TYPE "Warnungen"
TITLE =Warnmeldungen
AUTHOR : dfb
FAMILY : Meld
NAME : WarnMeld
VERSION : 0.1


  STRUCT
    Anzahl_Meldeworte : INT  := 12; // Anzahl Warnmeldeworte
HZ01 : STRUCT //Heizzone 01 Warnmeldungen 1-16
W001_HZ01_Brn_1_Stoer : Bool ;  //W001: Zone 1 Brenner 1 Brennerstörung
W002_HZ01_Brn_2_Stoer : Bool ;  //W002: Zone 1 Brenner 2 Brennerstörung
W003_HZ01_Brn_3_Stoer : Bool ;  //W003: Zone 1 Brenner 3 Brennerstörung
W004_HZ01_Brn_4_Stoer : Bool ;  //W004: Zone 1 Brenner 4 Brennerstörung
W005_HZ01_Brn_5_Stoer : Bool ;  //W005: Zone 1 Brenner 5 Brennerstörung
W006 : Bool ;  //W006:
W007 : Bool ;  //W007:
W008 : Bool ;  //W008:
W009 : Bool ;  //W009:
W010 : Bool ;  //W010:
W011 : Bool ;  //W011:
W012 : Bool ;  //W012:
W013 : Bool ;  //W013:
W014 : Bool ;  //W014:
W015 : Bool ;  //W015:
W016 : Bool ;  //W016:
END_STRUCT ;
HZ02 : STRUCT //Heizzone 02 Warnmeldungen 17-32
W017_HZ02_Brn_1_Stoer : Bool ;  //W017: Zone 2 Brenner 1 Brennerstörung
W018_HZ02_Brn_2_Stoer : Bool ;  //W018: Zone 2 Brenner 2 Brennerstörung
W019_HZ02_Brn_3_Stoer : Bool ;  //W019: Zone 2 Brenner 3 Brennerstörung
W020_HZ02_Brn_4_Stoer : Bool ;  //W020: Zone 2 Brenner 4 Brennerstörung
W021 : Bool ;  //W021:
W022 : Bool ;  //W022:
W023 : Bool ;  //W023:
W024 : Bool ;  //W024:
W025 : Bool ;  //W025:
W026 : Bool ;  //W026:
W027 : Bool ;  //W027:
W028 : Bool ;  //W028:
W029 : Bool ;  //W029:
W030 : Bool ;  //W030:
W031 : Bool ;  //W031:
W032 : Bool ;  //W032:
END_STRUCT ;
HZ03 : STRUCT //Heizzone 03 Warnmeldungen 33-48
W033_HZ03_Brn_1_Stoer : Bool ;  //W033: Zone 3 Brenner 1 Brennerstörung
W034_HZ03_Brn_2_Stoer : Bool ;  //W034: Zone 3 Brenner 2 Brennerstörung
W035_HZ03_Brn_3_Stoer : Bool ;  //W035: Zone 3 Brenner 3 Brennerstörung
W036 : Bool ;  //W036:
W037 : Bool ;  //W037:
W038 : Bool ;  //W038:
W039 : Bool ;  //W039:
W040 : Bool ;  //W040:
W041 : Bool ;  //W041:
W042 : Bool ;  //W042:
W043 : Bool ;  //W043:
W044 : Bool ;  //W044:
W045 : Bool ;  //W045:
W046 : Bool ;  //W046:
W047 : Bool ;  //W047:
W048 : Bool ;  //W048:
END_STRUCT ;
HZ04 : STRUCT //Heizzone 04 Warnmeldungen 49-64
W049_HZ04_Brn_1_Stoer : Bool ;  //W049: Zone 4 Brenner 1 Brennerstörung
W050_HZ04_Brn_2_Stoer : Bool ;  //W050: Zone 4 Brenner 2 Brennerstörung
W051 : Bool ;  //W051:
W052 : Bool ;  //W052:
W053 : Bool ;  //W053:
W054 : Bool ;  //W054:
W055 : Bool ;  //W055:
W056 : Bool ;  //W056:
W057 : Bool ;  //W057:
W058 : Bool ;  //W058:
W059 : Bool ;  //W059:
W060 : Bool ;  //W060:
W061 : Bool ;  //W061:
W062 : Bool ;  //W062:
W063 : Bool ;  //W063:
W064 : Bool ;  //W064:
END_STRUCT ;
HZ05 : STRUCT //Heizzone 05 Warnmeldungen 65-80
W065_HZ05_Brn_1_Stoer : Bool ;  //W065: Zone 5 Brenner 1 Brennerstörung
W066_HZ05_Brn_2_Stoer : Bool ;  //W066: Zone 5 Brenner 2 Brennerstörung
W067 : Bool ;  //W067:
W068 : Bool ;  //W068:
W069 : Bool ;  //W069:
W070 : Bool ;  //W070:
W071 : Bool ;  //W071:
W072 : Bool ;  //W072:
W073 : Bool ;  //W073:
W074 : Bool ;  //W074:
W075 : Bool ;  //W075:
W076 : Bool ;  //W076:
W077 : Bool ;  //W077:
W078 : Bool ;  //W078:
W079 : Bool ;  //W079:
W080 : Bool ;  //W080:
END_STRUCT ;
HZ06 : STRUCT //Heizzone 06 Warnmeldungen 81-96
W081_HZ06_Brn_1_Stoer : Bool ;  //W081: Zone 6 Brenner 1 Brennerstörung
W082_HZ06_Brn_2_Stoer : Bool ;  //W082: Zone 6 Brenner 2 Brennerstörung
W083_HZ06_Brn_3_Stoer : Bool ;  //W083: Zone 6 Brenner 3 Brennerstörung
W084 : Bool ;  //W084:
W085 : Bool ;  //W085:
W086 : Bool ;  //W086:
W087 : Bool ;  //W087:
W088 : Bool ;  //W088:
W089 : Bool ;  //W089:
W090 : Bool ;  //W090:
W091 : Bool ;  //W091:
W092 : Bool ;  //W092:
W093 : Bool ;  //W093:
W094 : Bool ;  //W094:
W095 : Bool ;  //W095:
W096 : Bool ;  //W096:
END_STRUCT ;
HZ07 : STRUCT //Heizzone 07 Warnmeldungen 97-112
W097_HZ07_Brn_1_Stoer : Bool ;  //W097: Zone 7 Brenner 1 Brennerstörung
W098_HZ07_Brn_2_Stoer : Bool ;  //W098: Zone 7 Brenner 2 Brennerstörung
W099 : Bool ;  //W099:
W100 : Bool ;  //W100:
W101 : Bool ;  //W101:
W102 : Bool ;  //W102:
W103 : Bool ;  //W103:
W104 : Bool ;  //W104:
W105 : Bool ;  //W105:
W106 : Bool ;  //W106:
W107 : Bool ;  //W107:
W108 : Bool ;  //W108:
W109 : Bool ;  //W109:
W110 : Bool ;  //W110:
W111 : Bool ;  //W111:
W112 : Bool ;  //W112:
END_STRUCT ;
NA_SK: STRUCT //Not Aus und Schutzkreise Meldungen 113-128
W113_Not_Aus_OE_ausgel : Bool ;  //W113: Not Aus hat ausgelöst
W114_Schkr_Ofeneinl : Bool ;  //W114: Schutzkreis Ofeneinlauf nicht geschlossen
W115_Schkr_Ofenausl : Bool ;  //W115: Schutzkreis Ofenauslauf nicht geschlossen
W116_NA_Tast_Ofeneinl : Bool ;  //W116: Not Aus Taster Bedienpult Ofeneinlauf betätigt
W117_NA_Tast_Ofenausl : Bool ;  //W117: Not Aus Taster Bedienpult Ofenauslauf betätigt
W118 : Bool ;  //W118:
W119 : Bool ;  //W119:
W120 : Bool ;  //W120:
W121 : Bool ;  //W121:
W122 : Bool ;  //W122:
W123 : Bool ;  //W123:
W124 : Bool ;  //W124:
W125 : Bool ;  //W125:
W126 : Bool ;  //W126:
W127 : Bool ;  //W127:
W128 : Bool ;  //W128:
END_STRUCT ;
Netz : STRUCT  //Versorgungsnetz Meldungen 129-144
W129_Q_Notnetz_niO : Bool ;  //W129: Hauptschalter Notnetz nicht eingeschaltet
W130_Notnetz_aktiv : Bool ;  //W130: Notstromversorgung aktiv
W131 : Bool ;  //W131:
W132 : Bool ;  //W132:
W133 : Bool ;  //W133:
W134 : Bool ;  //W134:
W135 : Bool ;  //W135:
W136 : Bool ;  //W136:
W137 : Bool ;  //W137:
W138 : Bool ;  //W138:
W139 : Bool ;  //W139:
W140 : Bool ;  //W140:
W141 : Bool ;  //W141:
W142 : Bool ;  //W142:
W143 : Bool ;  //W143:
W144 : Bool ;  //W144:
END_STRUCT ;
HZ08 : STRUCT //Heizzone 08 Warnmeldungen 145-160
W145_HZ08_Brn_1_Stoer : Bool ;  //W145: Zone 8 Brenner 1 Brennerstörung
W146_HZ08_Brn_2_Stoer : Bool ;  //W146: Zone 8 Brenner 2 Brennerstörung
W147 : Bool ;  //W147:
W148 : Bool ;  //W148:
W149 : Bool ;  //W149:
W150 : Bool ;  //W150:
W151 : Bool ;  //W151:
W152 : Bool ;  //W152:
W153 : Bool ;  //W153:
W154 : Bool ;  //W154:
W155 : Bool ;  //W155:
W156 : Bool ;  //W156:
W157 : Bool ;  //W157:
W158 : Bool ;  //W158:
W159 : Bool ;  //W159:
W160 : Bool ;  //W160:
END_STRUCT ;
HZ09 : STRUCT //Heizzone 09 Warnmeldungen 161-176
W161_HZ09_Brn_1_Stoer : Bool ;  //W161: Zone 9 Brenner 1 Brennerstörung
W162_HZ09_Brn_2_Stoer : Bool ;  //W162: Zone 9 Brenner 2 Brennerstörung
W163 : Bool ;  //W163:
W164 : Bool ;  //W164:
W165 : Bool ;  //W165:
W166 : Bool ;  //W166:
W167 : Bool ;  //W167:
W168 : Bool ;  //W168:
W169 : Bool ;  //W169:
W170 : Bool ;  //W170:
W171 : Bool ;  //W171:
W172 : Bool ;  //W172:
W173 : Bool ;  //W173:
W174 : Bool ;  //W174:
W175 : Bool ;  //W175:
W176 : Bool ;  //W176:
END_STRUCT ;
HZ10 : STRUCT //Heizzone 10 Warnmeldungen 177-192
W177_HZ10_Brn_1_Stoer : Bool ;  //W177: Zone 10 Brenner 1 Brennerstörung
W178_HZ10_Brn_2_Stoer : Bool ;  //W178: Zone 10 Brenner 2 Brennerstörung
W179 : Bool ;  //W179:
W180 : Bool ;  //W180:
W181 : Bool ;  //W181:
W182 : Bool ;  //W182:
W183 : Bool ;  //W183:
W184 : Bool ;  //W184:
W185 : Bool ;  //W185:
W186 : Bool ;  //W186:
W187 : Bool ;  //W187:
W188 : Bool ;  //W188:
W189 : Bool ;  //W189:
W190 : Bool ;  //W190:
W191 : Bool ;  //W191:
W192 : Bool ;  //W192:
END_STRUCT ;
END_STRUCT ;
END_TYPE
